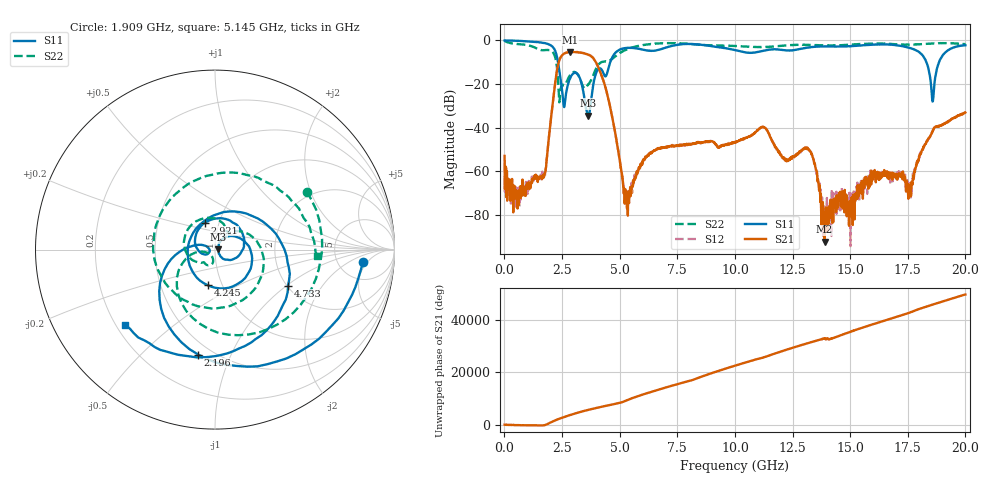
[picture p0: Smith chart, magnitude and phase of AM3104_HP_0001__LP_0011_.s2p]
!Created with skrf (http://scikit-rf.org).
# Hz S RI R 50.0
!freq ReS11 ImS11 ReS21 ImS21 ReS12 ImS12 ReS22 ImS22
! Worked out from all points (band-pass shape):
!   1601 points, 10 MHz to 20 GHz, reference 50 ohm
!   highest |S21| = -5.25 dB at 2.846 GHz (marker M1); lowest = -92.3 dB at 13.89 GHz (marker M2)
!   |S21| within 3 dB of the highest: 2.415 GHz to 3.863 GHz (1.449 GHz wide, 46.2 % of centre)
!   lowest |S11| = -34.4 dB at 3.646 GHz (marker M3), VSWR 1.04, Z = 51.9 + j0.256 ohm
!   |S11| at or under -10 dB: 2.327 GHz to 4.591 GHz (2.264 GHz wide, 65.4 % of centre); 18.31 GHz to 18.85 GHz (545.6 MHz wide, 2.94 % of centre)
!   |S22| runs from -28.4 to -0.2 dB; largest |S21 - S12| = 0.006
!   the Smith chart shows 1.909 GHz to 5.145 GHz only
!   S11 on the Smith chart (normalised r, x): 1.909 GHz: 8.86, -3.88; 2.196 GHz: 0.42, -0.76; 2.921 GHz: 0.86, +0.26; 4.245 GHz: 0.85, -0.35; 4.733 GHz: 2.02, -1.03; 5.145 GHz: 0.24, -0.35
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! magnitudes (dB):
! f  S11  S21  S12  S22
! 10 MHz  0.0  -52.9  -56.4  -0.2
! 672.2 MHz  -0.2  -70.6  -68.3  -1.7
! 1.697 GHz  -1.1  -62.0  -61.5  -4.5
! 1.909 GHz  -1.6  -46.8  -46.8  -4.4
! 2.196 GHz  -4.5  -20.1  -20.1  -7.5
! 2.571 GHz  -29.7  -6.2  -6.2  -20.4
! 2.846 GHz  -17.4  -5.2  -5.3  -15.9
! 2.921 GHz  -15.9  -5.3  -5.3  -14.9
! 3.346 GHz  -19.6  -5.6  -5.6  -19.4
! 3.646 GHz  -34.4  -6.6  -6.6  -20.2
! 4.245 GHz  -13.9  -16.9  -16.9  -9.9
! 4.733 GHz  -6.8  -38.1  -38.2  -8.0
! 5.145 GHz  -3.7  -65.2  -65.6  -4.9
! 5.37 GHz  -3.4  -69.2  -73.3  -3.8
! 6.682 GHz  -4.3  -49.6  -49.7  -1.3
! 10.01 GHz  -4.4  -46.6  -46.5  -2.5
! 13.34 GHz  -3.0  -52.3  -52.6  -2.1
! 13.89 GHz  -2.7  -92.3  -78.0  -2.2
! 16.68 GHz  -1.8  -63.5  -61.7  -1.5
! 17.6 GHz  -3.5  -71.4  -67.9  -1.9
! 18.58 GHz  -28.0  -41.8  -41.3  -1.4
! 20 GHz  -2.2  -33.1  -33.1  -1.7
